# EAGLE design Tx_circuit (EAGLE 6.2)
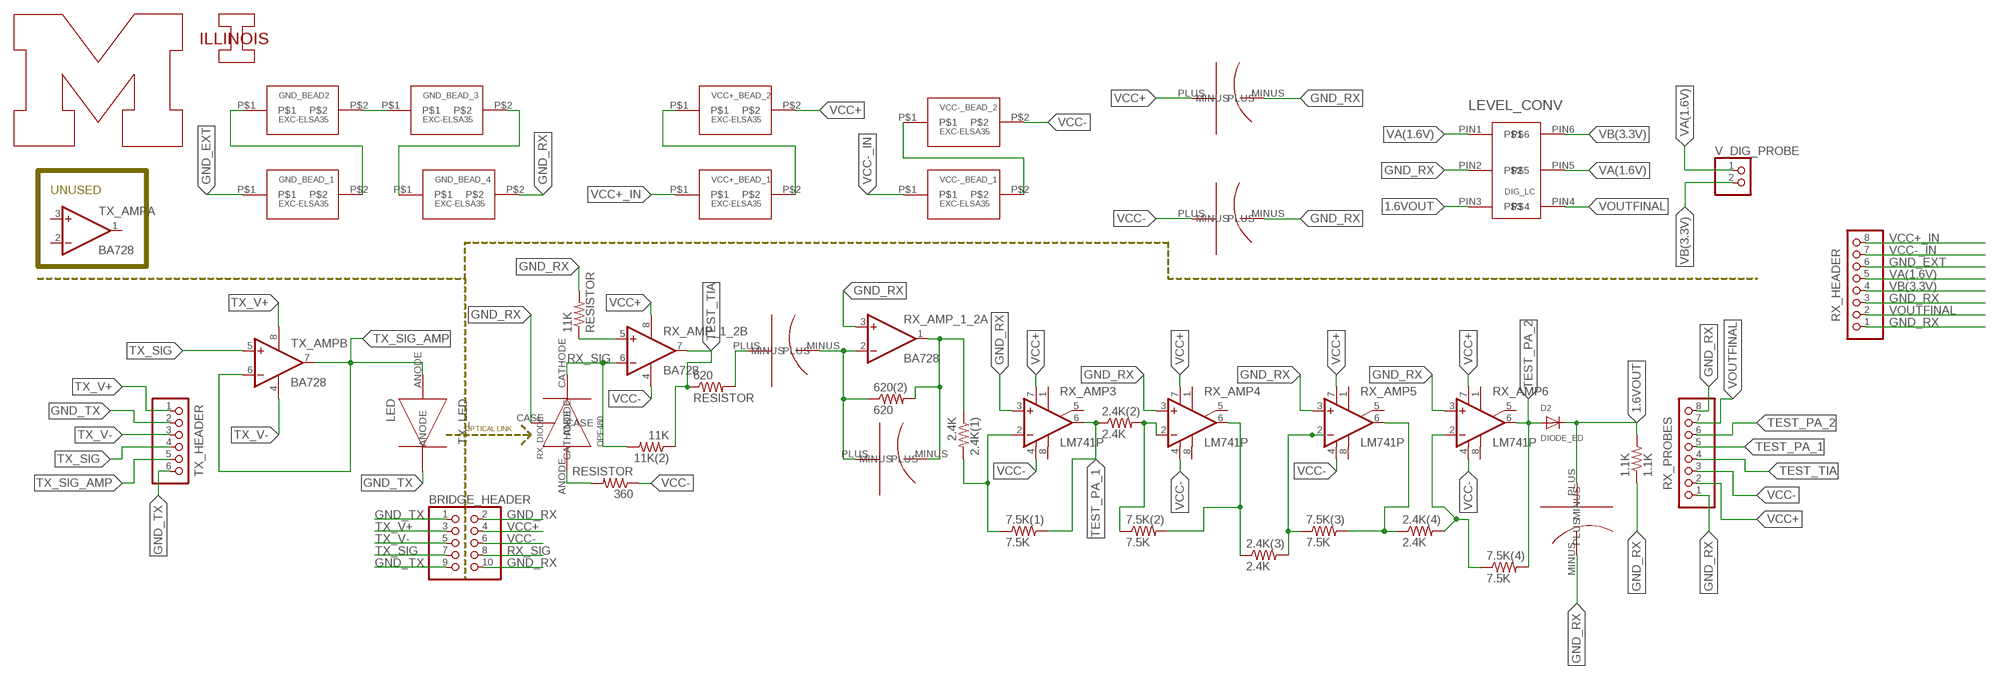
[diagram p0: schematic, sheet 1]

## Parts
1.1K  1.1K  RESISTOR  [R_US]
2.4K(1)  2.4K  RESISTOR  [R_US]
2.4K(2)  2.4K  RESISTOR  [R_US]
2.4K(3)  2.4K  RESISTOR  [R_US]
2.4K(4)  2.4K  RESISTOR  [R_US]
7.5K(1)  7.5K  RESISTOR  [R_US]
7.5K(2)  7.5K  RESISTOR  [R_US]
7.5K(3)  7.5K  RESISTOR  [R_US]
7.5K(4)  7.5K  RESISTOR  [R_US]
10PF  CAP_TINY  [FINAL_TINY_CAP]
11K  RESISTOR  [R_US]
11K(2)  11K  RESISTOR  [R_US]
100PF  100pF  CAP_TINY  [FINAL_TINY_CAP]
360  RESISTOR  [R_US]
620  RESISTOR  [R_US]
620(2)  620  RESISTOR  [R_US]
.1UF  CAP_.1F  [FINAL_SMALL_CAP]
BRIDGE_HEADER  PINHD-2X5  [2X05]
D2  DIODE_ED  DIODEDO-1N4148  [DO-1N4148]
DIG_LC  LEVEL_CONV  [SOT-23]
GND_BEAD2  EXC-ELSA35  [FB]
GND_BEAD_1  EXC-ELSA35  [FB]
GND_BEAD_3  EXC-ELSA35  [FB]
GND_BEAD_4  EXC-ELSA35  [FB]
RX_AMP3  LM741P  [DIL08]
RX_AMP4  LM741P  [DIL08]
RX_AMP5  LM741P  [DIL08]
RX_AMP6  LM741P  [DIL08]
RX_AMP_1_2  BA728  [DIL08]
RX_DIODE  OPF480  [PD]
RX_HEADER  PINHD-1X8  [1X08]
RX_PROBES  PINHD-1X8  [1X08]
TX_AMP  BA728  [DIL08]
TX_HEADER  PINHD-1X6  [1X06]
TX_LED  LED  [LED]
U$1  BLOCK_M1CM_TALL  [BLOCK_M_1CM]
U$2  BLOCK_I-ILLINOIS  [BLOCK-I_ILLINOIS]
V_DIG_PROBE  PINHD-1X2  [1X02]
VCC+_BEAD_1  EXC-ELSA35  [FB]
VCC+_BEAD_2  EXC-ELSA35  [FB]
VCC+_CAP  CAP_1000UF  [FINAL_LARGE_CAP]
VCC-_BEAD_1  EXC-ELSA35  [FB]
VCC-_BEAD_2  EXC-ELSA35  [FB]
VCC-_CAP  CAP_1000UF  [FINAL_LARGE_CAP]

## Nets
1.6VOUT: 1.1K.P$2 100PF.PLUS D2.C DIG_LC.PIN3
CAP-: 10PF.PLUS 620(2).P$1 .1UF.MINUS RX_AMP_1_2.2(A:-IN)
GND_EXT: GND_BEAD_1.P$1 RX_HEADER.6
GND_RX: 1.1K.P$1 11K.P$2 100PF.MINUS BRIDGE_HEADER.2 BRIDGE_HEADER.10 DIG_LC.PIN2 GND_BEAD_4.P$2 RX_AMP3.3(+IN) RX_AMP4.3(+IN) RX_AMP5.3(+IN) RX_AMP6.3(+IN) RX_AMP_1_2.3(A:+IN) RX_DIODE.CASE RX_HEADER.1 RX_HEADER.3 RX_PROBES.1 RX_PROBES.8 VCC+_CAP.MINUS VCC-_CAP.MINUS
GND_TX: BRIDGE_HEADER.1 BRIDGE_HEADER.9 TX_HEADER.2 TX_HEADER.6 TX_LED.CATHODE
N$5: 2.4K(3).P$2 7.5K(3).P$1 RX_AMP5.2(-IN)
N$6: 2.4K(4).P$1 7.5K(3).P$2 RX_AMP5.6(OUT)
N$7: 2.4K(4).P$2 7.5K(4).P$1 RX_AMP6.2(-IN)
N$9: 2.4K(1).P$2 7.5K(1).P$1 RX_AMP3.2(-IN)
N$11: 360.P$2 RX_DIODE.ANODE
N$13: 620.P$2 .1UF.PLUS
N$15: 2.4K(2).P$2 7.5K(2).P$1 RX_AMP4.2(-IN)
N$16: GND_BEAD2.P$1 GND_BEAD_1.P$2
N$17: GND_BEAD2.P$2 GND_BEAD_3.P$1
N$18: GND_BEAD_3.P$2 GND_BEAD_4.P$1
N$19: 11K.P$1 RX_AMP_1_2.5(B:+IN)
N$20: VCC+_BEAD_1.P$2 VCC+_BEAD_2.P$1
N$22: VCC-_BEAD_1.P$2 VCC-_BEAD_2.P$1
N$23: 2.4K(1).P$1 10PF.MINUS 620(2).P$2 RX_AMP_1_2.1(A:OUT)
N$31: 2.4K(3).P$1 7.5K(2).P$2 RX_AMP4.6(OUT)
RX_SIG: 11K(2).P$2 BRIDGE_HEADER.8 RX_AMP_1_2.6(B:-IN) RX_DIODE.CATHODE
TEST_PA_1: 2.4K(2).P$1 7.5K(1).P$2 RX_AMP3.6(OUT) RX_PROBES.5
TEST_PA_2: 7.5K(4).P$2 D2.A RX_AMP6.6(OUT) RX_PROBES.6
TEST_TIA: 11K(2).P$1 620.P$1 RX_AMP_1_2.7(B:OUT) RX_PROBES.4
TX_SIG: BRIDGE_HEADER.7 TX_AMP.5(B:+IN) TX_HEADER.4
TX_SIG_AMP: TX_AMP.6(B:-IN) TX_AMP.7(B:OUT) TX_HEADER.5 TX_LED.ANODE
TX_V+: BRIDGE_HEADER.3 TX_AMP.8(P:V+) TX_HEADER.1
TX_V-: BRIDGE_HEADER.5 TX_AMP.4(P:V-) TX_HEADER.3
VA(1.6V): DIG_LC.PIN1 DIG_LC.PIN5 RX_HEADER.5 V_DIG_PROBE.1
VB(3.3V): DIG_LC.PIN6 RX_HEADER.4 V_DIG_PROBE.2
VCC+: BRIDGE_HEADER.4 RX_AMP3.7(V+) RX_AMP4.7(V+) RX_AMP5.7(V+) RX_AMP6.7(V+) RX_AMP_1_2.8(P:V+) RX_PROBES.2 VCC+_BEAD_2.P$2 VCC+_CAP.PLUS
VCC+_IN: RX_HEADER.8 VCC+_BEAD_1.P$1
VCC-: 360.P$1 BRIDGE_HEADER.6 RX_AMP3.4(V-) RX_AMP4.4(V-) RX_AMP5.4(V-) RX_AMP6.4(V-) RX_AMP_1_2.4(P:V-) RX_PROBES.3 VCC-_BEAD_2.P$2 VCC-_CAP.PLUS
VCC-_IN: RX_HEADER.7 VCC-_BEAD_1.P$1
VOUTFINAL: DIG_LC.PIN4 RX_HEADER.2 RX_PROBES.7
Unconnected: RX_AMP3.1(ON1) RX_AMP3.5(ON2) RX_AMP3.8(OPT) RX_AMP4.1(ON1) RX_AMP4.5(ON2) RX_AMP4.8(OPT) RX_AMP5.1(ON1) RX_AMP5.5(ON2) RX_AMP5.8(OPT) RX_AMP6.1(ON1) RX_AMP6.5(ON2) RX_AMP6.8(OPT) TX_AMP.1(A:OUT) TX_AMP.2(A:-IN) TX_AMP.3(A:+IN)

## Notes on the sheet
- UNUSED
- OPTICAL LINK

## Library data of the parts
1.1K 2.4K(1) 2.4K(2) 2.4K(3) 2.4K(4) 7.5K(1) 7.5K(2) 7.5K(3) 7.5K(4) 11K 11K(2) 360 620 620(2) = VLClib:RESISTOR
10PF 100PF = VLClib:CAP_TINY
.1UF = VLClib:CAP_.1F
BRIDGE_HEADER = pinhead:PINHD-2X5: PIN HEADER
D2 = adafruit:DIODE: Diode
DIG_LC = VLClib:LEVEL_CONV
GND_BEAD2 GND_BEAD_1 GND_BEAD_3 GND_BEAD_4 VCC+_BEAD_1 VCC+_BEAD_2 VCC-_BEAD_1 VCC-_BEAD_2 = VLClib:EXC-ELSA35
RX_AMP3-RX_AMP6 = linear:*741: OP AMP
RX_AMP_1_2 TX_AMP = linear:BA728: Dual operational amplifier Source: ROHM BA728.pdf
RX_DIODE = VLClib:OPF480
RX_HEADER RX_PROBES = pinhead:PINHD-1X8: PIN HEADER
TX_HEADER = pinhead:PINHD-1X6: PIN HEADER
TX_LED = VLClib:LED
U$1 = umich:BLOCK_M
U$2 = umich:BLOCK_I-ILLINOIS
V_DIG_PROBE = pinhead:PINHD-1X2: PIN HEADER
VCC+_CAP VCC-_CAP = VLClib:CAP_1000UF

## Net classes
0 default: width 0.381 mm, drill 0.508 mm, clearance 0.254 mm

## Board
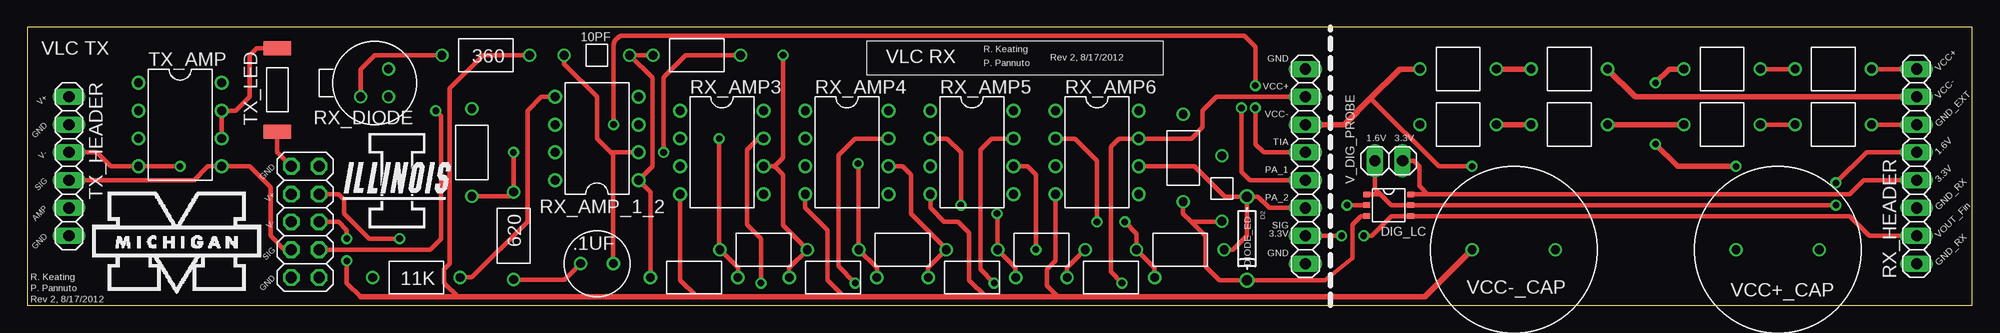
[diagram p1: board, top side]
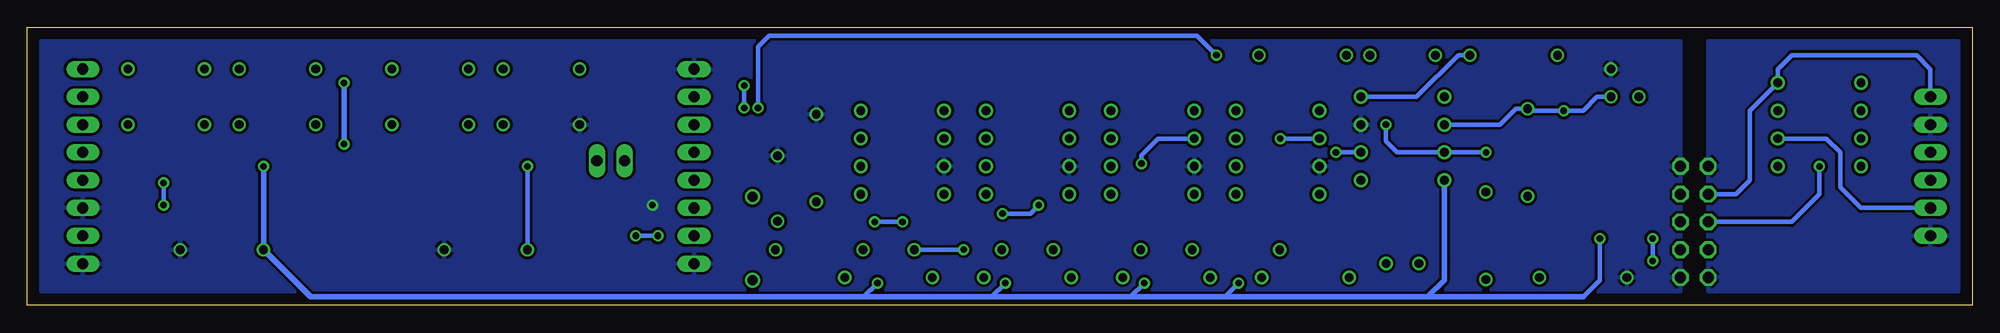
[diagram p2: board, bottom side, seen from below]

Size 177.8 x 25.4 mm. Coordinates in mm from the lower left corner, seen from the top.
Outline: 0,0 177.8,0 177.8,25.4 0,25.4 0,0
Copper layers (1*16): Top 0.0178mm / dielectric 59mil / Bottom 0.0178mm
Design rules: minimum track width 6mil, minimum drill 14mil, track to track 6mil, track to pad 6mil, pad to pad 6mil, via to via 6mil, smd to smd 6mil, copper to edge 20mil, drill to drill 16mil, minimum pad ring 8mil, minimum via ring 8mil, stop-mask expansion 3mil, vias tented up to drill 0mil, thermal gap 10mil

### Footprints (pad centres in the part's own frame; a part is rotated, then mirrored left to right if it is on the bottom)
R_US = drill 0.8: P$1 -4,0; P$2 4,0
FINAL_TINY_CAP = drill 0.8: MINUS 3,0; PLUS -3,0
FINAL_SMALL_CAP = drill 0.8: MINUS 0,-1.5; PLUS 0,1.5
2X05 = drill 1.016 octagon: 1 -5.08,-1.27; 2 -5.08,1.27; 3 -2.54,-1.27; 4 -2.54,1.27; 5 0,-1.27; 6 0,1.27; 7 2.54,-1.27; 8 2.54,1.27; 9 5.08,-1.27; 10 5.08,1.27
DO-1N4148 = drill 0.9: A -3.81,0; C 3.81,0
SOT-23 = smd 0.5 x 0.6: PIN1 -1,-2; PIN2 0,-2; PIN3 1,-2; PIN4 1,2; PIN5 0,2; PIN6 -1,2
FB = drill 0.8: P$1 -3.5,0; P$2 3.5,0
DIL08 = drill 0.813 pad 1.27: 1 -3.81,-3.81; 2 -1.27,-3.81; 3 1.27,-3.81; 4 3.81,-3.81; 5 3.81,3.81; 6 1.27,3.81; 7 -1.27,3.81; 8 -3.81,3.81
PD = drill 0.8: ANODE 1.27,-1.27; CASE -1.27,1.27; CATHODE 1.27,1.27
1X08 = drill 1.016 long: 1 -8.89,0; 2 -6.35,0; 3 -3.81,0; 4 -1.27,0; 5 1.27,0; 6 3.81,0; 7 6.35,0; 8 8.89,0
1X06 = drill 1.016 long: 1 -6.35,0; 2 -3.81,0; 3 -1.27,0; 4 1.27,0; 5 3.81,0; 6 6.35,0
LED = smd 1.27 x 2.54: ANODE -3.81,0; CATHODE 3.81,0
1X02 = drill 1.016 long: 1 -1.27,0; 2 1.27,0
FINAL_LARGE_CAP = drill 0.8: MINUS 0,-3.81; PLUS 0,3.81

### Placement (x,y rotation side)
1.1K  105.66,13.46 270 top
2.4K(1)  60.96,2.54 0 top
2.4K(2)  73.66,2.54 0 top
2.4K(3)  86.36,2.54 0 top
2.4K(4)  99.06,2.54 0 top
7.5K(1)  67.31,5.08 0 top
7.5K(2)  80.01,5.08 0 top
7.5K(3)  92.71,5.08 0 top
7.5K(4)  105.41,5.08 0 top
10PF  52.07,22.86 0 top
11K  35.56,2.54 180 top
11K(2)  40.64,13.97 90 top
100PF  109.22,10.67 90 top
360  41.91,22.86 180 top
620  44.45,6.35 270 top
620(2)  61.21,22.86 180 top
.1UF  52.07,3.81 90 top
BRIDGE_HEADER  25.4,7.62 270 top
D2  111.51,6.1 270 top
DIG_LC  124.46,9.14 270 top
GND_BEAD2  154.94,16.51 180 top
GND_BEAD_1  165.1,16.51 180 top
GND_BEAD_3  140.97,16.51 180 top
GND_BEAD_4  130.81,16.51 180 top
RX_AMP3  63.5,13.97 270 top
RX_AMP4  74.93,13.97 270 top
RX_AMP5  86.36,13.97 270 top
RX_AMP6  97.79,13.97 270 top
RX_AMP_1_2  52.07,15.24 90 top
RX_DIODE  31.75,20.32 270 top
RX_HEADER  172.72,12.7 90 top
RX_PROBES  116.84,12.7 270 top
TX_AMP  13.97,16.51 270 top
TX_HEADER  3.81,12.7 270 top
TX_LED  22.86,19.68 270 top
U$1  13.72,5.33 0 top
U$2  28.7,6.86 0 top
V_DIG_PROBE  124.46,13.21 0 top
VCC+_BEAD_1  165.1,21.59 180 top
VCC+_BEAD_2  154.94,21.59 180 top
VCC+_CAP  160.02,5.08 90 top
VCC-_BEAD_1  140.97,21.59 180 top
VCC-_BEAD_2  130.81,21.59 180 top
VCC-_CAP  135.89,5.08 90 top

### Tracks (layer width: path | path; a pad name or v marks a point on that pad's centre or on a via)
1.6VOUT
  Top 0.406: 1.1K.P$2 105.66,8.38 106.43,7.62 | 106.43,7.62 109.17,7.62 100PF.PLUS | 106.43,7.62 107.7,6.35 107.7,3.56 108.97,2.29 D2.C 118.62,2.29 121.16,4.32 121.16,7.37 121.92,8.13 122.44,8.13 DIG_LC.PIN3
CAP-  (via drill 0.6)
  Top 0.406: 10PF.PLUS 49.07,22.05 52.07,19.05 52.07,15.24 53.34,13.97 | 53.34,13.97 RX_AMP_1_2.2 | .1UF.MINUS 53.57,13.74 53.34,13.97 | v58.17,13.97 58.17,20.83 60.2,22.86 620(2).P$1
  Bottom 0.406: RX_AMP_1_2.2 v58.17,13.97
GND_EXT
  Top 0.406: GND_BEAD_1.P$1 RX_HEADER.6
GND_RX  (via drill 0.6)
  Top 0.406: DIG_LC.PIN2 v120.65,9.14
  pour Bottom: 26.67,24.13 176.53,24.13 176.53,1.27 26.67,1.27
GND_TX
  Top 0.406: TX_LED.CATHODE 22.86,13.97 BRIDGE_HEADER.1
  pour Bottom: 1.27,24.13 24.13,24.13 24.13,1.27 1.27,1.27
N$5  (via drill 0.6)
  Top 0.406: 2.4K(3).P$2 90.36,3.43 7.5K(3).P$1 88.71,8.32 v88.65,8.38 | v85.34,9.14 85.34,13.97 84.07,15.24 RX_AMP5.2
  Bottom 0.406: v88.65,8.38 86.11,8.38 v85.34,9.14
N$6  (via drill 0.6)
  Top 0.406: 2.4K(4).P$1 95.06,3.43 7.5K(3).P$2 | v92.2,5.08 92.2,11.94 91.44,12.7 RX_AMP5.6
  Bottom 0.406: 7.5K(3).P$2 v92.2,5.08
N$7  (via drill 0.6)
  Top 0.406: 2.4K(4).P$2 103.06,3.43 7.5K(4).P$1 101.41,6.54 v100.33,7.62 | v97.79,7.62 97.79,13.21 95.76,15.24 RX_AMP6.2
  Bottom 0.406: v100.33,7.62 v97.79,7.62
N$9  (via drill 0.6)
  Top 0.406: 2.4K(1).P$2 64.96,3.43 7.5K(1).P$1 63.25,5.14 v63.25,15.24
  Bottom 0.406: RX_AMP3.2 v63.25,15.24
N$11
  Top 0.406: 360.P$2 31.75,22.86 30.48,21.59 RX_DIODE.ANODE
N$13
  Top 0.406: 620.P$2 49.11,2.35 .1UF.PLUS
N$15  (via drill 0.6)
  Top 0.406: 2.4K(2).P$2 77.66,3.43 7.5K(2).P$1 76.01,12.89 v75.95,12.95
  Bottom 0.406: v75.95,12.95 75.95,13.72 74.42,15.24 RX_AMP4.2
N$16
  Top 0.406: GND_BEAD2.P$1 GND_BEAD_1.P$2
N$17
  Top 0.508: GND_BEAD2.P$2 GND_BEAD_3.P$1
N$18
  Top 0.508: GND_BEAD_3.P$2 GND_BEAD_4.P$1
N$19
  Top 0.406: 11K.P$1 40.64,2.54 45.72,7.62 45.72,17.78 46.99,19.05 RX_AMP_1_2.5
N$20
  Top 0.406: VCC+_BEAD_1.P$2 VCC+_BEAD_2.P$1
N$22
  Top 0.508: VCC-_BEAD_2.P$1 VCC-_BEAD_1.P$2
N$23
  Top 0.406: 620(2).P$2 10PF.MINUS 57.15,20.78 57.15,12.7 RX_AMP_1_2.1 56.96,10.35 2.4K(1).P$1
N$31
  Top 0.406: 2.4K(3).P$1 82.36,3.43 7.5K(2).P$2 84.01,5.14 80.77,8.38 80.77,11.94 80.01,12.7 RX_AMP4.6
RX_SIG  (via drill 0.6)
  Top 0.406: BRIDGE_HEADER.8 36.83,5.08 37.85,6.1 37.85,17.27 v37.34,17.78
  Bottom 0.406: RX_DIODE.CATHODE 34.29,19.05 35.56,17.78 36.83,17.78 v37.34,17.78 40.45,17.78 11K(2).P$2 41.72,17.97 43.18,16.51 RX_AMP_1_2.6
TEST_PA_1  (via drill 0.6)
  Top 0.406: 2.4K(2).P$1 69.66,3.43 7.5K(1).P$2 69.09,7.3 69.09,11.94 68.33,12.7 | RX_AMP3.6 68.33,12.7 | 68.33,12.7 69.09,13.46 v69.09,22.86 | RX_PROBES.5 111.76,11.43 111,12.19 v111,18.03
  Bottom 0.406: v69.09,22.86 70.87,24.64 109.98,24.64 111,23.62 v111,18.03
TEST_PA_2
  Top 0.406: RX_AMP6.6 106.68,12.7 109.47,9.91 D2.A | D2.A 112.52,9.91 113.54,8.89 RX_PROBES.6 | 7.5K(4).P$2 110.24,5.08 111.51,6.35 D2.A
TEST_TIA  (via drill 0.6)
  Top 0.406: 11K(2).P$1 44.07,9.97 620.P$1 v44.45,13.97 | v53.59,16.51 53.59,23.88 arc-60 54.36,24.64 111.25,24.64 112.27,23.62 v112.27,20.07 | RX_PROBES.4 113.03,13.97 112.27,14.73 v112.27,18.03
  Bottom 0.406: v44.45,13.97 RX_AMP_1_2.7 52.58,13.97 53.59,14.99 v53.59,16.51 | v112.27,18.03 v112.27,20.07
TX_SIG
  Top 0.406: BRIDGE_HEADER.7 23.5,5.08 22.23,6.35 22.23,10.79 20.32,12.7 TX_AMP.5 16.51,12.7 15.24,11.43 TX_HEADER.4
TX_SIG_AMP
  Top 0.406: TX_LED.ANODE 20.95,23.5 20.32,22.86 20.32,19.05 19.05,17.78 TX_AMP.7 TX_AMP.6
  Bottom 0.406: TX_HEADER.5 10.16,8.89 12.06,10.79 12.06,13.97 13.34,15.24 TX_AMP.6
TX_V+
  Bottom 0.406: TX_HEADER.1 3.81,21.59 5.08,22.86 16.51,22.86 17.78,21.59 TX_AMP.8 20.32,17.78 20.32,11.43 21.59,10.16 BRIDGE_HEADER.3
TX_V-  (via drill 0.6)
  Top 0.406: v13.97,12.7 TX_AMP.4 7.62,12.7 6.35,13.97 TX_HEADER.3
  Bottom 0.406: v13.97,12.7 13.97,10.16 16.51,7.62 BRIDGE_HEADER.5
VA(1.6V)  (via drill 0.6)
  Top 0.406: v165.35,9.14 DIG_LC.PIN5 124.71,9.14 123.71,10.14 | v165.35,11.18 168.15,13.97 RX_HEADER.5 | DIG_LC.PIN1 123.71,10.14 | V_DIG_PROBE.1 123.19,10.67 123.71,10.14
  Bottom 0.406: v165.35,9.14 v165.35,11.18
VB(3.3V)
  Top 0.406: DIG_LC.PIN6 128.02,10.14 | 128.02,10.14 166.61,10.14 167.89,11.43 RX_HEADER.4 | V_DIG_PROBE.2 126.75,13.21 127.25,12.7 127.25,10.91 128.02,10.14
VCC+  (via drill 0.6)
  Top 0.406: RX_AMP3.7 66.8,15.24 65.79,14.22 65.79,7.37 67.06,6.1 v67.06,2.03 | v75.69,2.03 74.17,3.56 74.17,13.72 75.69,15.24 RX_AMP4.7 | RX_AMP5.7 88.14,15.24 87.12,14.22 87.12,3.3 v88.39,2.03 | v100.08,2.03 99.06,3.05 99.06,14.48 99.82,15.24 RX_AMP6.7 106.43,15.24 107.44,16.26 107.44,17.78 108.71,19.05 RX_PROBES.2 | v34.04,6.1 31.24,6.1 28.96,8.38 28.96,9.65 28.45,10.16 BRIDGE_HEADER.4
  Top 0.508: v156.21,12.7 150.88,12.7 v148.84,14.73 | v148.84,20.32 150.11,21.59 VCC+_BEAD_2.P$2
  Bottom 0.406: v88.39,2.03 89.66,0.76 | v100.08,2.03 101.35,0.76 | v75.69,2.03 76.96,0.76 | v67.06,2.03 68.33,0.76 | 35.56,0.76 34.04,2.29 v34.04,6.1
  Bottom 0.508: 49.78,0.76 68.33,0.76 76.96,0.76 89.66,0.76 101.35,0.76 151.89,0.76 VCC+_CAP.PLUS v156.21,12.7 | RX_AMP_1_2.8 48.26,2.29 49.78,0.76 | v148.84,14.73 v148.84,20.32 | 49.78,0.76 35.56,0.76
VCC+_IN
  Top 0.406: VCC+_BEAD_1.P$1 RX_HEADER.8
VCC-  (via drill 0.6)
  Top 0.406: 360.P$1 41.66,22.86 38.61,19.81 38.61,3.81 38.1,3.3 38.1,2.03 39.37,0.76 | RX_AMP3.4 59.69,2.29 61.21,0.76 | RX_AMP4.4 71.12,8.89 73.15,6.86 73.15,2.29 74.68,0.76 | RX_AMP5.4 82.55,8.89 83.82,7.62 85.09,7.62 86.11,6.6 86.11,2.29 87.63,0.76 | RX_AMP6.4 93.98,4.06 93.22,3.3 93.22,1.78 94.23,0.76 | v132.08,12.7 129.03,12.7 122.81,18.92 | 30.48,0.76 29.21,2.03 v29.21,4.06 | v29.21,6.1 29.21,6.86 28.45,7.62 BRIDGE_HEADER.6
  Top 0.508: 30.48,0.76 39.37,0.76 61.21,0.76 74.68,0.76 87.63,0.76 94.23,0.76 127.76,0.76 VCC-_CAP.PLUS | RX_PROBES.3 120.4,16.51 122.81,18.92 125.48,21.59 VCC-_BEAD_2.P$2
  Bottom 0.406: 360.P$1 46.99,22.86 50.8,19.05 RX_AMP_1_2.4 | VCC-_CAP.PLUS v132.08,12.7 | v29.21,4.06 v29.21,6.1
VCC-_IN
  Top 0.508: RX_HEADER.7 147.01,19.05 VCC-_BEAD_1.P$1
VOUTFINAL  (via drill 0.6)
  Top 0.406: RX_HEADER.2 168.4,6.35 166.61,8.14 DIG_LC.PIN4 126.44,8.13 124.71,8.13 122.94,6.35 v122.17,6.35 | RX_PROBES.7 v120.14,6.35
  Bottom 0.406: v120.14,6.35 v122.17,6.35

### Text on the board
tPlace: VLC TX | R. Keating | GND | VLC RX | P. Pannuto | Rev 2, 8/17/2012 | VCC+ | VCC+ | V+ | VCC- | VCC- | GND | GND_EXT | TIA | 1.6V | 3.3V | V- | 1.6V | GND | PA_1 | SIG | 3.3V | V+ | PA_2 | AMP | GND_RX | V- | SIG | GND | 3.3V | VOUT_Fin | SIG | GND | GND_RX | GND | R. Keating | P. Pannuto | Rev 2, 8/17/2012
